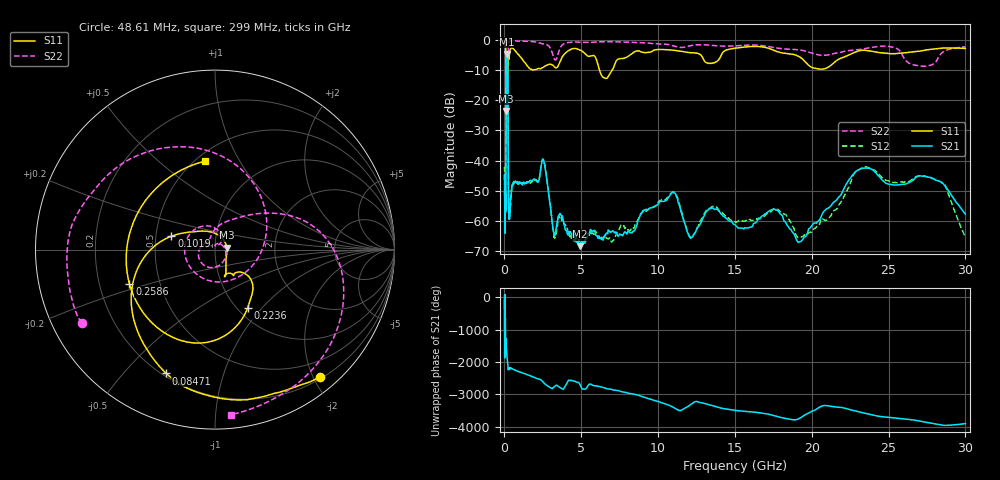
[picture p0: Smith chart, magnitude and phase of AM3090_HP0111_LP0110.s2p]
! Date/Time: Thu, Feb 28, 2019 2:01 PM
! Network Analyzer: Agilent Technologies E8364B Rev: A.07.50.67
! Sweep from 0.010 to 30.000 GHz, 1601 Points, Sweep Type: LOG
! Power Supply: 5.023 V, 0.002 A
# Hz S DB R 50
!freq MagS11 AngS11 MagS21 AngS21 MagS12 AngS12 MagS22 AngS22
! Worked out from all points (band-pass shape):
!   1601 points, 10 MHz to 30 GHz, reference 50 ohm
!   highest |S21| = -4.63 dB at 159.1 MHz (marker M1); lowest = -68.4 dB at 4.927 GHz (marker M2)
!   |S21| within 3 dB of the highest: 113.6 MHz to 211.8 MHz (98.21 MHz wide, 60.4 % of centre)
!   lowest |S11| = -23.6 dB at 109.9 MHz (marker M3), VSWR 1.14, Z = 57 + j1.14 ohm
!   |S11| at or under -10 dB: 100.8 MHz to 214.1 MHz (113.3 MHz wide, 72 % of centre); 6.184 GHz to 7.012 GHz (827.7 MHz wide, 12.5 % of centre)
!   |S22| runs from -33.9 to -0.2 dB; largest |S21 - S12| = 0.013
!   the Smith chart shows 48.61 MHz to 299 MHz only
!   S11 on the Smith chart (normalised r, x): 48.61 MHz: 0.23, -2.11; 84.71 MHz: 0.22, -0.66; 101.9 MHz: 0.60, +0.10; 223.6 MHz: 1.11, -0.84; 258.6 MHz: 0.33, -0.17; 299 MHz: 0.56, +0.73
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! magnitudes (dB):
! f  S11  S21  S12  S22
! 10 MHz  -0.3  -46.3  -42.6  -0.6
! 38.04 MHz  -0.5  -60.2  -60.6  -1.4
! 48.61 MHz  -0.7  -51.5  -51.9  -1.5
! 84.71 MHz  -2.6  -53.5  -55.4  -5.3
! 101.9 MHz  -11.9  -17.1  -17.1  -15.2
! 109.9 MHz  -23.6  -9.1  -9.1  -15.9
! 144.7 MHz  -16.4  -4.8  -4.7  -27.7
! 159.1 MHz  -16.0  -4.6  -4.6  -21.5
! 223.6 MHz  -8.5  -11.9  -11.9  -11.4
! 258.6 MHz  -5.8  -51.6  -51.5  -1.6
! 299 MHz  -6.1  -56.8  -55.1  -0.7
! 550.5 MHz  -2.8  -47.7  -47.9  -0.3
! 2.084 GHz  -9.8  -46.8  -46.6  -0.7
! 2.533 GHz  -9.0  -39.8  -39.7  -1.3
! 3.236 GHz  -8.8  -64.8  -65.5  -6.3
! 4.927 GHz  -3.4  -68.4  -66.5  -0.8
! 7.926 GHz  -5.8  -64.0  -62.6  -0.7
! 10.81 GHz  -3.3  -51.1  -51.0  -1.7
! 12.13 GHz  -4.2  -65.8  -65.5  -1.9
! 19.7 GHz  -7.9  -64.3  -64.6  -3.9
! 23.59 GHz  -3.5  -42.5  -42.1  -2.7
! 30 GHz  -2.8  -57.8  -65.5  -2.3
